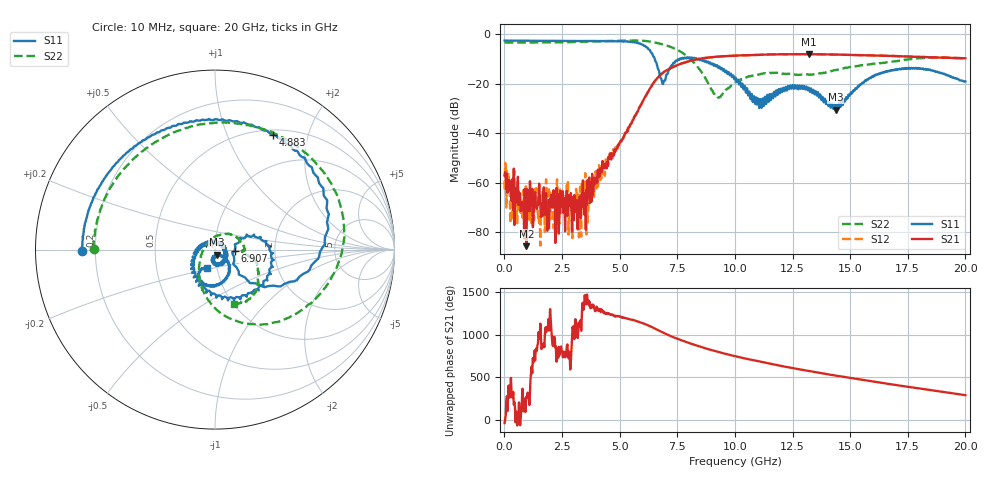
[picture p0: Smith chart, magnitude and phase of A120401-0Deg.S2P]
!  2-Port S-parameters saved by WinCal
! VAR MeasName=S-Parameters (CALIBRATED_DATA) read from VNA (N5244A)
! VAR MeasDate=11/21/2012 9:53:38 AM
! VAR NAME=A120401-0Deg
! VAR FILENAME=A120401-0Deg.S2P
! VAR DATE=11/21/2012 9:53:38 AM
! VAR PHYS_PORTS=1,2
# Hz S MA R 50
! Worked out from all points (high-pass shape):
!   801 points, 10 MHz to 20 GHz, reference 50 ohm
!   highest |S21| = -8.09 dB at 13.23 GHz (marker M1); lowest = -85.7 dB at 959.5 MHz (marker M2)
!   |S21| within 3 dB of the highest: 7.955 GHz to end of sweep
!   lowest |S11| = -30.5 dB at 14.38 GHz (marker M3), VSWR 1.06, Z = 50.9 - j2.86 ohm
!   |S11| at or under -10 dB: 6.521 GHz to 7.613 GHz (1.091 GHz wide, 15.4 % of centre); 8.354 GHz to 8.428 GHz (74.38 MHz wide, 0.886 % of centre); 8.432 GHz to end of sweep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
!   |S22| runs from -25.6 to -2.6 dB; largest |S21 - S12| = 0.0037
!   S11 on the Smith chart (normalised r, x): 10 MHz: 0.15, -0.01; 4.883 GHz: 0.56, +1.47; 6.907 GHz: 1.24, -0.02; 20 GHz: 0.90, -0.18
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1e7  0.7414 -179.3  0.001406 -38.0  0.0007308 69.3  0.6738 179.6
9.59525e8  0.7369 161.4  5.187e-05 -95.2  0.0001445 -81.9  0.6753 156.8
1.084462e9  0.7345 159.0  0.0002591 175.6  0.0001605 38.7  0.6765 153.8
1.834088e9  0.7317 144.0  0.0003795 11.6  0.0004325 132.8  0.6772 135.8
2.483762e9  0.73 130.4  0.0005231 100.2  0.0003642 -15.3  0.6843 119.7
3.083462e9  0.7268 116.7  0.0002577 105.6  0.0004001 -43.6  0.695 104.6
3.358325e9  0.7236 109.9  0.0005985 147.9  0.0009231 -74.9  0.7014 97.8
4.882562e9  0.7159 63.3  0.004966 141.2  0.00538 141.7  0.7334 53.9
5.90705e9  0.6417 10.3  0.03583 67.0  0.03646 68.8  0.7374 17.3
6.681662e9  0.1919 -46.3  0.1374 -25.9  0.1371 -25.8  0.6542 -17.6
6.90655e9  0.1093 -3.5  0.1697 -55.6  0.1702 -55.6  0.6149 -28.5
7.431288e9  0.2904 9.4  0.2289 -117.2  0.2288 -117.2  0.5007 -56.1
8.255875e9  0.3227 -43.0  0.3035 162.4  0.3027 162.5  0.2556 -102.9
9.255375e9  0.2212 -106.5  0.3511 81.6  0.35 81.7  0.05256 143.8
1.0005e10  0.1285 -163.0  0.3672 30.3  0.3671 30.3  0.1049 57.1
1.105448e10  0.03207 83.6  0.3818 -32.6  0.3829 -32.7  0.1532 12.6
1.322839e10  0.07483 -88.6  0.3939 -145.7  0.3941 -145.8  0.1519 -2.7
1.335332e10  0.06438 -97.7  0.3923 -151.7  0.3931 -151.8  0.1527 -4.2
1.437781e10  0.02973 -71.1  0.3864 161.0  0.3867 160.9  0.1887 -9.8
1.667666e10  0.1783 -72.4  0.3625 63.0  0.3641 62.7  0.2749 -27.6
1.827586e10  0.1958 -112.5  0.3434 -1.2  0.3445 -1.0  0.3312 -49.7
2e10  0.1105 -114.4  0.3245 -68.9  0.3246 -68.9  0.3216 -70.7
